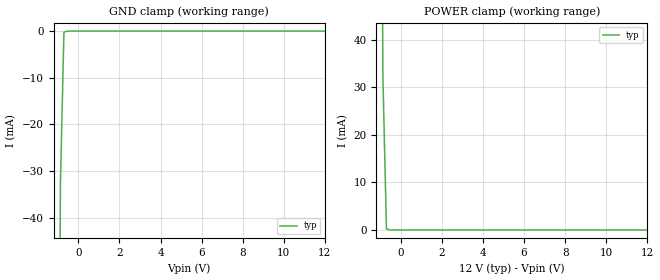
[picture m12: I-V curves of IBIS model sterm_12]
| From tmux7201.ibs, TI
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| sterm_12
[Model]   sterm_12
Model_type   Terminator
|   typ   min   max
C_comp   2.533030e-11   NA   NA
[Voltage Range]   12   NA   NA
[Temperature Range]   27   NA   NA
[Power Clamp Reference]   12   NA   NA
[GND Clamp Reference]   0   NA   NA
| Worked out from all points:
|   GND clamp passes 1 mA (typ) near -0.71 V on its own axis
|   POWER clamp passes 1 mA (typ) near -0.71 V on its own axis
[GND Clamp]
|   Voltage   I(typ)   I(min)   I(max)
-5V       -9.926A    NA         NA
-1.051V   -178.1mA   NA         NA
-878.8mV  -32.8mA    NA         NA
-707.1mV  -233uA     NA         NA
-535.4mV  -609.2nA   NA         NA
12V       472.1pA    NA         NA
[POWER Clamp]
|   Voltage   I(typ)   I(min)   I(max)
-5V       13.26A     NA         NA
-1.05V    174.4mA    NA         NA
-878.8mV  32.16mA    NA         NA
-707.1mV  229.2uA    NA         NA
-535.4mV  537.6nA    NA         NA
12V       -472.7pA   NA         NA
